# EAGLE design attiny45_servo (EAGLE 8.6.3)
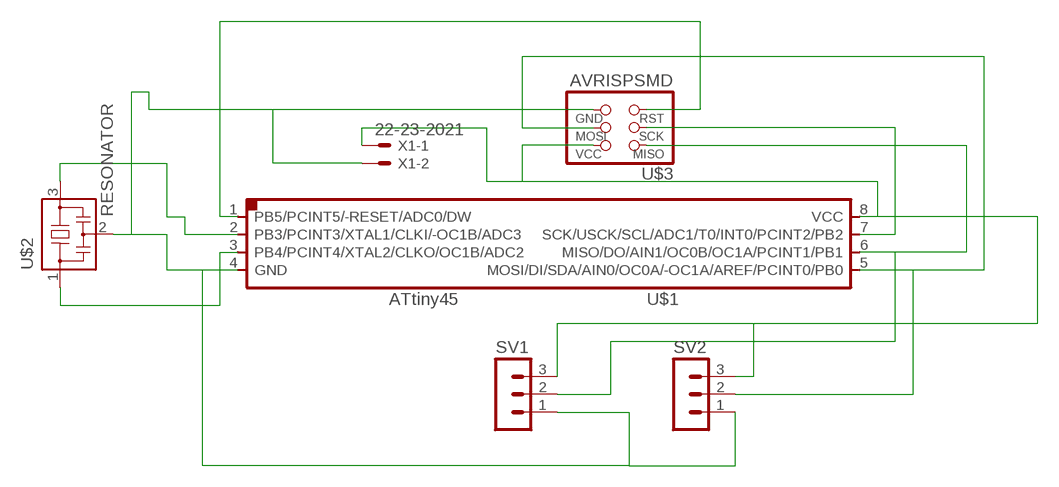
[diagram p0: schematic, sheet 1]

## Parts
SV1  MA03-1  [MA03-1]
SV2  MA03-1  [MA03-1]
U$1  ATTINY45SI  [SOIC8]
U$2  RESONATOR  [EFOBM]
U$3  AVRISPSMD  [2X03SMD]
X1  22-23-2021  [22-23-2021]

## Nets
N$3: U$1.2(PB3/PCINT3/XTAL1/CLKI/-OC1B/ADC3) U$2.3
N$4: SV1.2 U$1.6(MISO/DO/AIN1/OC0B/OC1A/PCINT1/PB1) U$3.1(MISO)
N$5: SV2.2 U$1.5(MOSI/DI/SDA/AIN0/OC0A/-OC1A/AREF/PCINT0/PB0) U$3.4(MOSI)
N$7: U$1.7(SCK/USCK/SCL/ADC1/T0/INT0/PCINT2/PB2) U$3.3(SCK)
N$8: U$1.1(PB5/PCINT5/-RESET/ADC0/DW) U$3.5(RST)
N$9: U$1.3(PB4/PCINT4/XTAL2/CLKO/OC1B/ADC2) U$2.1
N$10: SV1.3 SV2.3 U$1.8(VCC) U$3.2(VCC) X1.1
N$11: SV1.1 SV2.1 U$1.4(GND) U$2.2 U$3.6(GND) X1.2

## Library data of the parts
SV1 SV2 = con-lstb:MA03-1: PIN HEADER; OC_FARNELL: unknown; OC_NEWARK: unknown
U$1 = fab:ATTINY45
U$2 = fab:RESONATOR
U$3 = fab:AVRISP
X1 = con-molex:22-23-2021: .100" (2.54mm) Center Header - 2 Pin; MF: MOLEX; MPN: 22-23-2021; OC_FARNELL: 1462926; OC_NEWARK: 25C3832

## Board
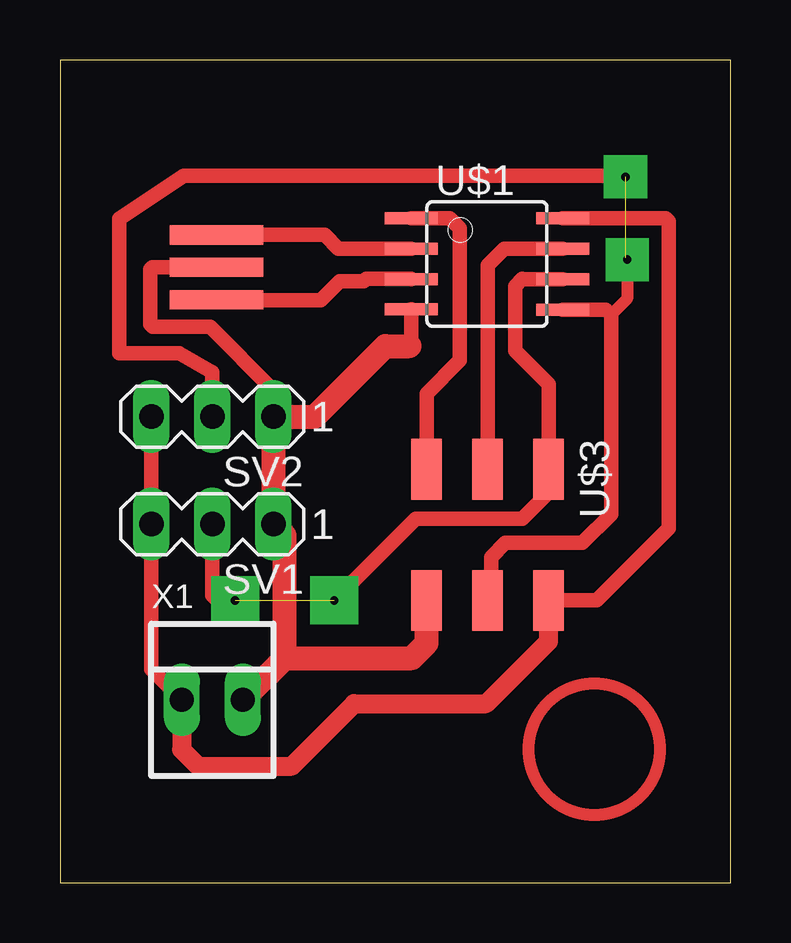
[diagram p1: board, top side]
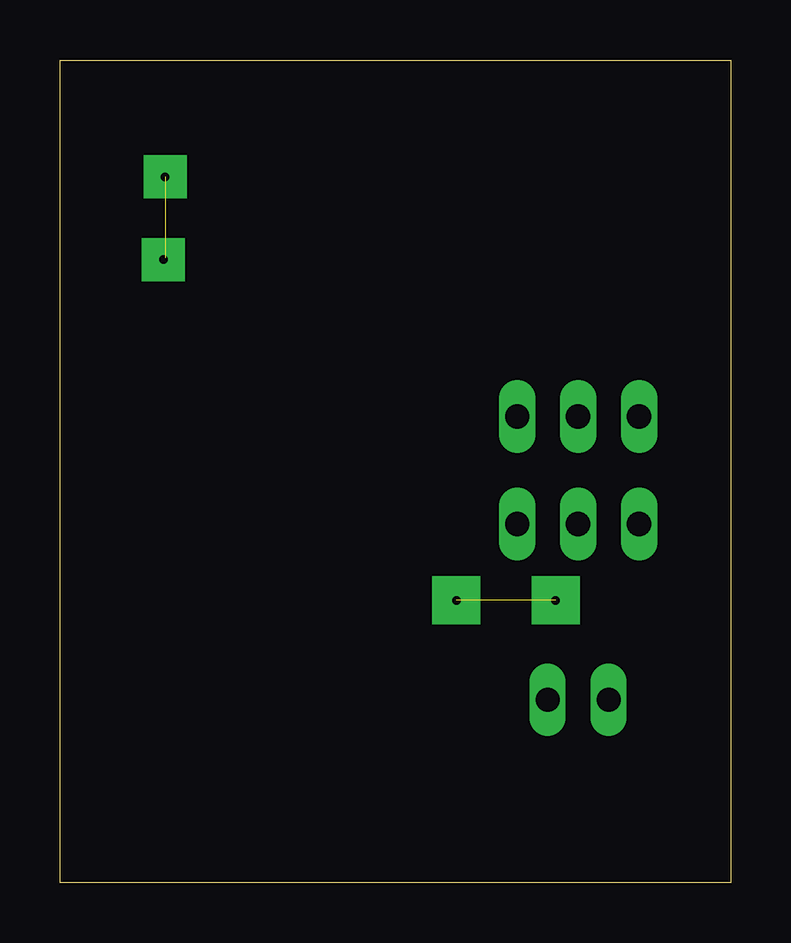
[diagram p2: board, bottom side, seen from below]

Size 27.94 x 34.28 mm. Coordinates in mm from the lower left corner, seen from the top.
Outline: 0,0 27.94,0 27.94,34.28 0,34.28 0,0
Copper layers (1*16): Top 0.035mm / dielectric 1.5mm / Bottom 0.035mm
Design rules "default": minimum track width 6mil, minimum drill 0.35mm, track to track 6mil, track to pad 6mil, pad to pad 6mil, via to via 6mil, smd to smd 6mil, copper to edge 40mil, drill to drill 6mil, minimum pad ring 10mil, minimum via ring 8mil, stop-mask expansion 4mil, vias tented up to drill 0mil, thermal gap 10mil

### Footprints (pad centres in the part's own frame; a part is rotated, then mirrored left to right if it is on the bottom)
MA03-1 = drill 1.016 long: 1 -2.54,0; 2 0,0; 3 2.54,0
SOIC8 = smd 0.5 x 2.2: 1 -1.905,-3.154; 2 -0.645,-3.154; 3 0.625,-3.154; 4 1.895,-3.154; 5 1.905,3.154; 6 0.635,3.154; 7 -0.635,3.154; 8 -1.905,3.154
EFOBM = smd 0.8 x 3.9: 1 -1.35,0; 2 0,0; 3 1.35,0
2X03SMD = smd 2.54 x 1.27: 1 -2.54,2.54; 2 2.92,2.54; 3 -2.54,0; 4 2.92,0; 5 -2.54,-2.54; 6 2.92,-2.54
22-23-2021 = drill 1 long: 1 -1.27,0; 2 1.27,0

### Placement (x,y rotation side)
SV1  6.35,14.94 180 top
SV2  6.35,19.42 180 top
U$1  17.79,25.78 270 top
U$2  6.52,25.64 90 top
U$3  17.82,14.68 270 top
X1  6.35,7.62 0 top

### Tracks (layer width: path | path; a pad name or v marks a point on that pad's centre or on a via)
N$3
  Top 0.6: U$2.3 11.03,26.99 11.6,26.42 U$1.2
N$4  (via drill 0.35 pad 2)  (1 unrouted)
  Top 0.6: U$1.6 19.27,25.14 19.26,25.16 18.96,24.86 18.96,22.16 20.36,20.76 U$3.1 20.36,16.26 19.26,15.16 14.83,15.16 v11.43,11.76 | SV1.2 6.35,11.97 6.56,11.76 v7.29,11.76
N$5  (via drill 0.35 pad 1.8)  (1 unrouted)
  Top 0.5: 23.86,29.46 23.81,29.41 v23.56,29.41 | v23.63,25.96 23.63,24.34 22.96,23.66
  Top 0.6: U$3.4 17.96,11.9 17.96,13.56 18.56,14.16 21.76,14.16 22.96,15.36 22.96,23.66 22.74,23.88 U$1.5 | SV2.2 6.35,21.27 4.96,22.06 2.46,22.06 2.46,27.66 5.16,29.46 23.86,29.46
  Bottom 0.5: 23.56,26.03 v23.63,25.96
N$7
  Top 0.6: U$1.7 18.52,26.41 17.82,25.72 U$3.3
N$8
  Top 0.6: U$1.1 16.23,27.68 16.66,27.26 16.66,21.76 15.28,20.38 U$3.5
N$9
  Top 0.6: U$2.1 6.55,24.26 10.86,24.26 11.66,25.06 12.66,25.06 12.76,25.16 U$1.3
N$10
  Top 0.6: U$1.8 25.23,27.68 25.36,27.56 25.36,14.76 22.36,11.76 U$3.2 | X1.1 3.81,8.89 SV1.3 SV2.3
  Top 0.8: X1.1 5.08,5.58 5.06,5.56 5.76,4.86 9.66,4.86 12.26,7.46 17.76,7.46 20.36,10.06 U$3.2
N$11
  Top 0.6: U$2.2 3.84,25.64 3.76,25.56 3.76,23.26 3.86,23.16 6.26,23.16 8.89,20.53 SV2.1 | 14.56,22.36 14.64,22.44 U$1.4
  Top 1: X1.2 9.36,9.36 | 9.36,9.36 14.66,9.36 15.28,9.98 U$3.6 | 9.36,9.36 9.36,14.47 SV1.1 SV2.1 10.62,19.42 13.56,22.36 14.56,22.36
(copper drawn outside any net)
  shapes: Top circle x1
